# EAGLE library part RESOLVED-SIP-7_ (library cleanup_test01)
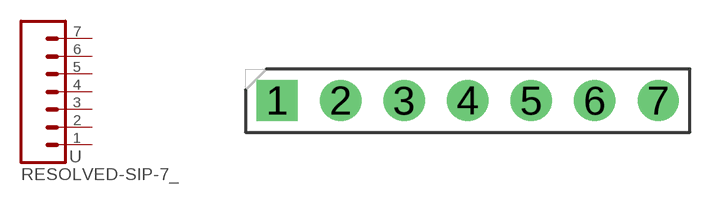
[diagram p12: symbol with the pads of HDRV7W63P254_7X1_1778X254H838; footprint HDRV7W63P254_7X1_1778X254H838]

Designator prefix -

## RESOLVED-SIP-7_2.54-SPACE-VERTICAL  [HDRV7W63P254_7X1_1778X254H838]
1  1  pas
2  2  pas
3  3  pas
4  4  pas
5  5  pas
6  6  pas
7  7  pas

## Footprint HDRV7W63P254_7X1_1778X254H838 (pad centres in mm)
drill 1.1 pad 1.65 square: 1 0,0
drill 1.1 pad 1.65: 2 2.54,0; 3 5.08,0; 4 7.62,0; 5 10.16,0; 6 12.7,0; 7 15.24,0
